DATA_BLOCK "Db_DataForDCS"
TITLE =
VERSION : 0.1


  STRUCT
   PressureTank_S1 : REAL ;	//PRESSURE INDICATOR 004600VA002A (0-16 bar) S1 - EW30 - 6005004600PT015
   PressureTank_S2 : REAL ;	//PRESSURE INDICATOR 004600VA002B (0-16 bar) S2 - EW32 - 6005004600PT016
   PressureTank_S3 : REAL ;	//PRESSURE INDICATOR 004600VA003 (0-16 bar) S3 - EW34 - 6005004600PT017
   PressureTank_S4 : REAL ;	//PRESSURE INDICATOR
   TemperatureTank_S1 : REAL ;	//TEMPERATURE INDICATOR 004600VA002A (0-60 °C) S1 - EW40 - 6005004600TT002
   TemperatureTank_S2 : REAL ;	//TEMPERATURE INDICATOR 004600VA002B (0-60 °C) S2 - EW42 - 6005004600TT003
   TemperatureTank_S3 : REAL ;	//TEMPERATURE INDICATOR 004600VA003 ((0-60 °C) S3 - EW44 - 6005004600TT004
   TemperatureTank_S4 : REAL ;	//TEMPERATURE INDICATOR
   HumidutyLine : REAL ;	//HUMIDUTY INDICATOR - EW52 - 6005004600AT001
   PressureLine : REAL ;	//PRESSURE INDICATOR LINE 004600IA046-2"-A55-N  (0-16 bar)-EW50 - 6005004600PT014
   FlowLine : REAL ;	//FLOW INDICATOR - EW54 - 6005004600FT001
   TemperatureComp_A : REAL ;	//TEMPERATURE INDICATOR COMPRESSOR A - 6005004600TT010A
   PressureComp_A : REAL ;	//PRESSURE INDICATOR COMPRESSOR A - 6005004600PT011A
   TemperatureComp_B : REAL ;	//TEMPERATURE INDICATOR COMPRESSOR B -6005004600TT010B
   PressureComp_B : REAL ;	//PRESSURE INDICATOR COMPRESSOR B - 6005004600PT011B
   TemperatureComp_C : REAL ;	//TEMPERATURE INDICATOR COMPRESSOR C - 6005004600TT010B
   PressureComp_C : REAL ;	//PRESSURE INDICATOR COMPRESSOR C -6005004600PT011B
   T6005004600UY007 : INT ;	//CLOSE VALVE UV007 FOR LOW PRES.(6barg)-6005004600UY007
   T6005004600ZLH007 : INT ;	//VALVE UV007 OPEN - 6005004600ZLH007
   T6005004600ZLL007 : INT ;	//VALVE UV007 CLOSE - 6005004600ZLL007
   T6005004600UL101 : INT ;	//COLUMN A ON LINE  - 6005004600UL101
   T6005004600UL102 : INT ;	//COLUMN A REGENERETING  - 6005004600UL102
   T6005004600UL108 : INT ;	//COLUMN A RE-PRESSURING - 6005004600UL108
   T6005004600UL109 : INT ;	//COLUMN A STAND BY - 6005004600UL109
   T6005004600UL115 : INT ;	//COLUMN B ON LINE  - 6005004600UL115
   T6005004600UL116 : INT ;	//COLUMN B REGENERETING  - 6005004600UL116
   T6005004600UL122 : INT ;	//COLUMN B RE-PRESSURING - 6005004600UL122
   T6005004600UL123 : INT ;	//COLUMN B STAND BY - 6005004600UL123
   T6005004600UA130 : INT ;	//DEW POINT ALARM - 6005004600UA130
   T6005004600UA136 : INT ;	//SENSOR ERROR - 6005004600UA136
   T6005004600UL137 : INT ;	//SERVICE INTERVAL - 6005004600UL137
   T6005004600UL111 : INT ;	//FAULT RELAY ACTIVE - 6005004600UL111
   T6005004600UL201 : INT ;	//COLUMN A ON LINE  - 6005004600UL201
   T6005004600UL202 : INT ;	//COLUMN A REGENERETING  - 6005004600UL202
   T6005004600UL208 : INT ;	//COLUMN A RE-PRESSURING - 6005004600UL208
   T6005004600UL209 : INT ;	//COLUMN A STAND BY - 6005004600UL209
   T6005004600UL215 : INT ;	//COLUMN B ON LINE  - 6005004600UL215
   T6005004600UL216 : INT ;	//COLUMN B REGENERETING  - 6005004600UL216
   T6005004600UL222 : INT ;	//COLUMN B REPRESSURING - 6005004600UL222
   T6005004600UL223 : INT ;	//COLUMN B STAND BY - 6005004600UL223
   T6005004600UA230 : INT ;	//DEW POINT ALARM - 6005004600UA230
   T6005004600UA236 : INT ;	//SENSOR ERROR - 6005004600UA236
   T6005004600UL237 : INT ;	//SERVICE INTERVAL - 6005004600UL237
   T6005004600UL211 : INT ;	//FAULT RELAY ACTIVE - 6005004600UL211
   T6005004600UL301 : INT ;	//COLUMN A ON LINE  - 6005004600UL301
   T6005004600UL302 : INT ;	//COLUMN A REGENERETING  - 6005004600UL302
   T6005004600UL308 : INT ;	//COLUMN A RE-PRESSURING - 6005004600UL308
   T6005004600UL309 : INT ;	//COLUMN A STAND BY - 6005004600UL309
   T6005004600UL315 : INT ;	//COLUMN B ON LINE  - 6005004600UL315
   T6005004600UL316 : INT ;	//COLUMN B REGENERETING  - 6005004600UL316
   T6005004600UL322 : INT ;	//COLUMN B REPRESSURING - 6005004600UL322
   T6005004600UL323 : INT ;	//COLUMN B STAND BY - 6005004600UL323
   T6005004600UA330 : INT ;	//DEW POINT ALARM - 6005004600UA330
   T6005004600UA336 : INT ;	//SENSOR ERROR - 6005004600UA336
   T6005004600UL337 : INT ;	//SERVICE INTERVAL - 6005004600UL337
   T6005004600UL311 : INT ;	//FAULT RELAY ACTIVE - 6005004600UL311
   T6005004600UL001A : INT ;	//RUN / STOP COMPRESSOR A - 6005004600UL001A
   T6005004600UL002A : INT ;	//LOAD / UNLOAD COMPRESSOR A  - 6005004600UL002A
   T6005004600UA003A : INT ;	//GENERAL WARNING COMPRESSOR A  - 6005004600UA003A
   T6005004600UA012A : INT ;	//SENSOR ERROR COMPRESSOR A  - 6005004600UA012A
   T6005004600UL001B : INT ;	//RUN / STOP COMPRESSOR B - 6005004600UL001B
   T6005004600UL002B : INT ;	//LOAD / UNLOAD COMPRESSOR B - 6005004600UL002B
   T6005004600UA003B : INT ;	//GENERAL WARNING COMPRESSOR B - 6005004600UA003B
   T6005004600UA012B : INT ;	//SENSOR ERROR COMPRESSOR B - 6005004600UA012B
   T6005004600UL001C : INT ;	//RUN / STOP COMPRESSOR C - 6005004600UL001C
   T6005004600UL002C : INT ;	//LOAD / UNLOAD COMPRESSOR C - 6005004600UL002C
   T6005004600UA003C : INT ;	//GENERAL WARNING COMPRESSOR C - 6005004600UA003C
   T6005004600UA012C : INT ;	//SENSOR ERROR COMPRESSOR C - 6005004600UA012C
   OverrideDewPoint : INT ;	//OVERRIDE DEW POINT
   StartStop_Dryer1 : INT ;	//START STOP DRYER 1; 0:= STOP 1:=START
   StartStop_Dryer2 : INT ;	//START STOP DRYER 2; 0:= STOP 1:=START
   StartStop_Dryer3 : INT ;	//START STOP DRYER 3; 0:= STOP 1:=START
   AutoDryer_1 : INT ;	//MANUAL AUTO DRYER 1;0:= MANUAL 1:=AUTO
   AutoDryer_2 : INT ;	//MANUAL AUTO DRYER 1;0:= MANUAL 2:=AUTO
   AutoDryer_3 : INT ;	//MANUAL AUTO DRYER 1;0:= MANUAL 3:=AUTO
   AlarmLevelSwitch : INT ;	//ALARM LEVEL SWITCH
   ShutDownCompressor_1 : INT ;	//SHUT DOWN COMPRESSOR 1;0:= NOT SHUT DOWN 1:=SHUT DOWN
   ShutDownCompressor_2 : INT ;	//SHUT DOWN COMPRESSOR 2;0:= NOT SHUT DOWN 1:=SHUT DOWN
   ShutDownCompressor_3 : INT ;	//SHUT DOWN COMPRESSOR 3;0:= NOT SHUT DOWN 1:=SHUT DOWN
   PDP_Essiccatore_Comp_A : INT ;	//DEW POINT COMPRESSOR 1 PDP
   PDP_Essiccatore_Comp_B : INT ;	//DEW POINT COMPRESSORE 2 PDP
   PDP_Essiccatore_Comp_C : INT ;	//DEW POINT COMPRESSORE 3 PDP
   AirEnvironment_Comp_A : INT ;	//ARI ENVIRONMENT COMPRESSOR 1
   AirEnvironment_Comp_B : INT ;	//ARI ENVIRONMENT COMPRESSOR 2
   AirEnvironment_Comp_C : INT ;	//ARI ENVIRONMENT COMPRESSOR 3
   CompA_MotorDryer : INT ;	//COMPRESSOR A MOTOR DRYER
   CompB_MotorDryer : INT ;	//COMPRESSOR B MOTOR DRYER
   CompC_MotorDryer : INT ;	//COMPRESSOR C MOTOR DRYER
   CompA_EnableMotorPrinc : INT ;	//COMPRESSOR A ENABLE FRIST MOTOR
   CompB_EnableMotorPrinc : INT ;	//COMPRESSOR B ENABLE FRIST MOTOR
   CompC_EnableMotorPrinc : INT ;	//COMPRESSOR C ENABLE FRIST MOTOR
   CompA_AutomaticFunction : INT ;	//COMPRESSOR A AUTOMATIC MODE
   CompB_AutomaticFunction : INT ;	//COMPRESSOR B AUTOMATIC MODE
   CompC_AutomaticFunction : INT ;	//COMPRESSOR C AUTOMATIC MODE
   CompA_GeneralWarning : INT ;	//COMPRESSOR A GENERAL WARNING
   CompB_GeneralWarning : INT ;	//COMPRESSOR B GENERAL WARNING
   CompC_GeneralWarning : INT ;	//COMPRESSOR C GENERAL WARNING
   CompA_StopGeneralSec : INT ;	//COMPRESSOR A STOP GENERAL SECURITY
   CompB_StopGeneralSec : INT ;	//COMPRESSOR B STOP GENERAL SECURITY
   CompC_StopGeneralSec : INT ;	//COMPRESSOR C STOP GENERAL SECURITY
   CompA_HourFunction : INT ;	//COMPRESSOR A HOUR FUNCTION
   CompB_HourFunction : INT ;	//COMPRESSOR B HOUR FUNCTION
   CompC_HourFunction : INT ;	//COMPRESSOR C HOUR FUNCTION
   CompA_StartupMotor : INT ;	//COMPRESSOR A STARTUP MOTOR
   CompB_StartupMotor : INT ;	//COMPRESSOR B STARTUP MOTOR
   CompC_StartupMotor : INT ;	//COMPRESSOR C STARTUP MOTOR
   CompA_StartupDryer : INT ;	//COMPRESSOR A STARTUP DRYER
   CompB_StartupDryer : INT ;	//COMPRESSOR B STARTUP DRYER
   CompC_StartupDryer : INT ;	//COMPRESSOR C STARTUP DRYER
   CompA_ProtDewPoint : INT ;	//COMPRESSOR A PROTECTION DEW POINT
   CompB_ProtDewPoint : INT ;	//COMPRESSOR B PROTECTION DEW POINT
   CompC_ProtDewPoint : INT ;	//COMPRESSOR C PROTECTION DEW POINT
   CompA_NotCeckValidPress : INT ;	//COMPRESSOR A NOT CECK VALID PRESSURE
   CompB_NotCeckValidPress : INT ;	//COMPRESSOR B NOT CECK VALID PRESSURE
   CompC_NotCeckValidPress : INT ;	//COMPRESSOR C NOT CECK VALID PRESSURE
   CompA_WarningAdaptMot_1 : INT ;	//COMPRESSOR A WARNING ADAPTER MOTOR 1
   CompB_WarningAdaptMot_1 : INT ;	//COMPRESSOR B WARNING ADAPTER MOTOR 1
   CompC_WarningAdaptMot_1 : INT ;	//COMPRESSOR C WARNING ADAPTER MOTOR 1
   CompA_ProtFreezingDryer : INT ;	//COMPRESSOR A PROTECTION FREEZING DRYER
   CompB_ProtFreezingDryer : INT ;	//COMPRESSOR B PROTECTION FREEZING DRYER
   CompC_ProtFreezingDryer : INT ;	//COMPRESSOR C PROTECTION FREEZING DRYER
   Comp_A_MachineControMode : INT ;	//COMPRESSOR A MACHINE CONTROL MODE
   Comp_B_MachineControMode : INT ;	//COMPRESSOR B MACHINE CONTROL MODE
   Comp_C_MachineControMode : INT ;	//COMPRESSOR C MACHINE CONTROL MODE
   Comp_A_MachineMeccState : INT ;	//COMPRESSOR A MACHINE MECCANICAL STATE
   Comp_B_MachineMeccState : INT ;	//COMPRESSOR B MACHINE MECCANICAL STATE
   Comp_C_MachineMeccState : INT ;	//COMPRESSOR C MACHINE MECCANICAL STATE
   CompA_GeneralStatus : INT ;	//COMPRESSOR A GENERAL STATUS
   CompB_GeneralStatus : INT ;	//COMPRESSOR B GENERAL STATUS
   CompC_GeneralStatus : INT ;	//COMPRESSOR C GENERAL STATUS
  END_STRUCT ;
BEGIN
   PressureTank_S1 := 0.000000e+000;
   PressureTank_S2 := 0.000000e+000;
   PressureTank_S3 := 0.000000e+000;
   PressureTank_S4 := 0.000000e+000;
   TemperatureTank_S1 := 0.000000e+000;
   TemperatureTank_S2 := 0.000000e+000;
   TemperatureTank_S3 := 0.000000e+000;
   TemperatureTank_S4 := 0.000000e+000;
   HumidutyLine := 0.000000e+000;
   PressureLine := 0.000000e+000;
   FlowLine := 0.000000e+000;
   TemperatureComp_A := 0.000000e+000;
   PressureComp_A := 0.000000e+000;
   TemperatureComp_B := 0.000000e+000;
   PressureComp_B := 0.000000e+000;
   TemperatureComp_C := 0.000000e+000;
   PressureComp_C := 0.000000e+000;
   T6005004600UY007 := 0;
   T6005004600ZLH007 := 0;
   T6005004600ZLL007 := 0;
   T6005004600UL101 := 0;
   T6005004600UL102 := 0;
   T6005004600UL108 := 0;
   T6005004600UL109 := 0;
   T6005004600UL115 := 0;
   T6005004600UL116 := 0;
   T6005004600UL122 := 0;
   T6005004600UL123 := 0;
   T6005004600UA130 := 0;
   T6005004600UA136 := 0;
   T6005004600UL137 := 0;
   T6005004600UL111 := 0;
   T6005004600UL201 := 0;
   T6005004600UL202 := 0;
   T6005004600UL208 := 0;
   T6005004600UL209 := 0;
   T6005004600UL215 := 0;
   T6005004600UL216 := 0;
   T6005004600UL222 := 0;
   T6005004600UL223 := 0;
   T6005004600UA230 := 0;
   T6005004600UA236 := 0;
   T6005004600UL237 := 0;
   T6005004600UL211 := 0;
   T6005004600UL301 := 0;
   T6005004600UL302 := 0;
   T6005004600UL308 := 0;
   T6005004600UL309 := 0;
   T6005004600UL315 := 0;
   T6005004600UL316 := 0;
   T6005004600UL322 := 0;
   T6005004600UL323 := 0;
   T6005004600UA330 := 0;
   T6005004600UA336 := 0;
   T6005004600UL337 := 0;
   T6005004600UL311 := 0;
   T6005004600UL001A := 0;
   T6005004600UL002A := 0;
   T6005004600UA003A := 0;
   T6005004600UA012A := 0;
   T6005004600UL001B := 0;
   T6005004600UL002B := 0;
   T6005004600UA003B := 0;
   T6005004600UA012B := 0;
   T6005004600UL001C := 0;
   T6005004600UL002C := 0;
   T6005004600UA003C := 0;
   T6005004600UA012C := 0;
   OverrideDewPoint := 0;
   StartStop_Dryer1 := 0;
   StartStop_Dryer2 := 0;
   StartStop_Dryer3 := 0;
   AutoDryer_1 := 0;
   AutoDryer_2 := 0;
   AutoDryer_3 := 0;
   AlarmLevelSwitch := 0;
   ShutDownCompressor_1 := 0;
   ShutDownCompressor_2 := 0;
   ShutDownCompressor_3 := 0;
   PDP_Essiccatore_Comp_A := 0;
   PDP_Essiccatore_Comp_B := 0;
   PDP_Essiccatore_Comp_C := 0;
   AirEnvironment_Comp_A := 0;
   AirEnvironment_Comp_B := 0;
   AirEnvironment_Comp_C := 0;
   CompA_MotorDryer := 0;
   CompB_MotorDryer := 0;
   CompC_MotorDryer := 0;
   CompA_EnableMotorPrinc := 0;
   CompB_EnableMotorPrinc := 0;
   CompC_EnableMotorPrinc := 0;
   CompA_AutomaticFunction := 0;
   CompB_AutomaticFunction := 0;
   CompC_AutomaticFunction := 0;
   CompA_GeneralWarning := 0;
   CompB_GeneralWarning := 0;
   CompC_GeneralWarning := 0;
   CompA_StopGeneralSec := 0;
   CompB_StopGeneralSec := 0;
   CompC_StopGeneralSec := 0;
   CompA_HourFunction := 0;
   CompB_HourFunction := 0;
   CompC_HourFunction := 0;
   CompA_StartupMotor := 0;
   CompB_StartupMotor := 0;
   CompC_StartupMotor := 0;
   CompA_StartupDryer := 0;
   CompB_StartupDryer := 0;
   CompC_StartupDryer := 0;
   CompA_ProtDewPoint := 0;
   CompB_ProtDewPoint := 0;
   CompC_ProtDewPoint := 0;
   CompA_NotCeckValidPress := 0;
   CompB_NotCeckValidPress := 0;
   CompC_NotCeckValidPress := 0;
   CompA_WarningAdaptMot_1 := 0;
   CompB_WarningAdaptMot_1 := 0;
   CompC_WarningAdaptMot_1 := 0;
   CompA_ProtFreezingDryer := 0;
   CompB_ProtFreezingDryer := 0;
   CompC_ProtFreezingDryer := 0;
   Comp_A_MachineControMode := 0;
   Comp_B_MachineControMode := 0;
   Comp_C_MachineControMode := 0;
   Comp_A_MachineMeccState := 0;
   Comp_B_MachineMeccState := 0;
   Comp_C_MachineMeccState := 0;
   CompA_GeneralStatus := 0;
   CompB_GeneralStatus := 0;
   CompC_GeneralStatus := 0;
END_DATA_BLOCK

